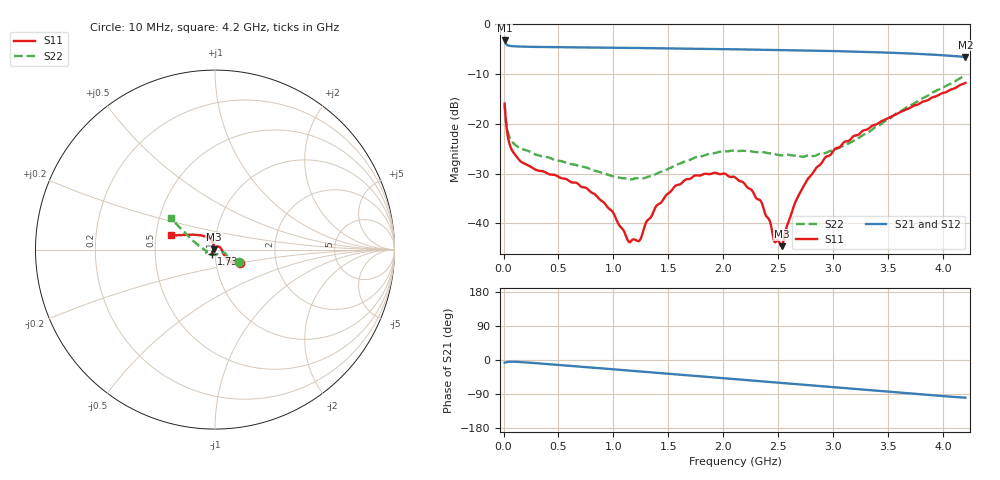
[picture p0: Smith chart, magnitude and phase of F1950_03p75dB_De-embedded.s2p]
! Integrated Device Technology
! Corporate Headquarters
! 6024 Silver Creek Valley Road
! San Jose, CA 95138  USA
! Phone:  1-408-284-8200
! Toll Free:  1-800-223-1366
! Webpage:  http://www.idt.com/
! Timing and RF Division
! 515 Groton Road, Suite 102
! Westford, MA 01886-6024
! Device:  F1950
! Description: 7-bit 0.25 dB Digital Step Attenuator
! Frequency:  150.0 -  4000.00 MHz
! Package:  4x4 mm Thin QFN Plastic Package: 24 pin
! Ports:  2 RF, 12 DC
!  Pin  1  = D0
!  Pin  2  = VDD
!  Pin  3  = Vmode
!  Pin  4  = GND
!  Pin  5  = RF1  =  Port 1
!  Pin  6  = GND
!  Pin  7  = GND
!  Pin  8  = GND
!  Pin  9  = GND
!  Pin 10  = GND
!  Pin 11  = GND
!  Pin 12  = GND
!  Pin 13  = GND
!  Pin 14  = RF2  =  Port 2
!  Pin 15  = GND
!  Pin 16  = LE
!  Pin 17  = CLK
!  Pin 18  = DATE
!  Pin 19  = D6
!  Pin 20  = D5
!  Pin 21  = D4
!  Pin 22  = D3
!  Pin 23  = D2
!  Pin 24  = D1
! State:  15
! Atten State:  3.75 dB
! Voltage:  +5.00 Volts
! Current:  Not Measured mA
! Data:  The device was measured on a the F195X evaluation board which has
!  individual transmission lines to the RF pins.  Data was collected
!  using a calibrated network analyzer.  The evaluation board was
!  de-embedded using a TRL calibration technique.
!  The reference plane is the edge of the package pin.
! Misc:  Board 2019
!  Action Tracker AT0250
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# GHz S dB R 50
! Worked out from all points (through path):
!   420 points, 10 MHz to 4.2 GHz, reference 50 ohm
!   highest |S21| = -3.28 dB at 10 MHz (marker M1); lowest = -6.6 dB at 4.2 GHz (marker M2)
!   group delay of S21, straight-line fit = 65.2 ps
!   lowest |S11| = -44.6 dB at 2.53 GHz (marker M3), VSWR 1.01, Z = 49.5 + j0.245 ohm
!   |S11| at or under -10 dB: start of sweep to end of sweep
!   |S22| runs from -31.2 to -10.3 dB; largest |S21 - S12| = 0.00073
!   S11 on the Smith chart (normalised r, x): 10 MHz: 1.31, -0.21; 1.73 GHz: 0.96, -0.04; 4.2 GHz: 0.60, +0.10
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0.01  -15.94 -28.7  -3.28 -6.7  -3.28 -6.7  -16.32 -27.0
0.06  -24.45 -31.1  -4.37 -4.5  -4.37 -4.5  -22.92 -26.1
0.15  -27.44 -14.6  -4.50 -5.3  -4.50 -5.3  -24.84 -18.9
0.71  -32.65 47.6  -4.68 -17.8  -4.68 -17.8  -28.59 -31.2
0.98  -37.37 73.4  -4.74 -24.1  -4.74 -24.1  -30.45 -53.8
1.15  -43.77 123.6  -4.78 -28.1  -4.78 -28.1  -31.15 -77.6
1.24  -43.32 172.2  -4.80 -30.2  -4.80 -30.2  -30.97 -90.3
1.3  -39.65 -163.4  -4.81 -31.6  -4.81 -31.6  -30.73 -100.9
1.41  -36.10 -146.1  -4.84 -34.2  -4.84 -34.2  -29.82 -115.9
1.56  -32.51 -136.1  -4.88 -37.7  -4.88 -37.7  -28.35 -131.8
1.73  -30.50 -129.0  -4.93 -41.7  -4.93 -41.7  -26.88 -144.2
1.92  -29.84 -123.9  -4.99 -46.2  -4.98 -46.2  -25.88 -153.4
2.11  -30.81 -121.0  -5.05 -50.6  -5.05 -50.7  -25.46 -158.5
2.34  -35.51 -127.4  -5.13 -56.0  -5.13 -56.1  -25.64 -162.2
2.42  -39.41 -138.9  -5.17 -57.9  -5.16 -57.9  -25.92 -162.6
2.46  -43.53 -155.7  -5.17 -58.8  -5.17 -58.8  -26.06 -162.8
2.53  -44.56 155.3  -5.20 -60.5  -5.20 -60.5  -26.31 -164.7
2.66  -35.42 109.8  -5.25 -63.6  -5.25 -63.6  -26.36 -166.1
2.81  -29.96 104.1  -5.31 -67.2  -5.31 -67.2  -26.47 -170.3
3.1  -23.63 115.0  -5.46 -74.2  -5.45 -74.3  -24.34 179.6
3.51  -18.72 136.1  -5.73 -84.1  -5.72 -84.2  -18.98 161.4
4.2  -11.80 161.7  -6.59 -99.4  -6.58 -99.5  -10.34 144.1
